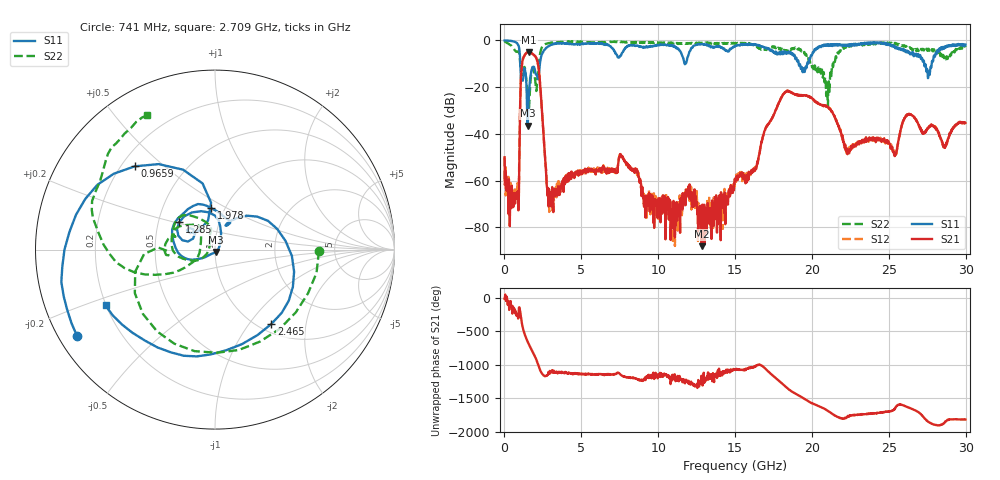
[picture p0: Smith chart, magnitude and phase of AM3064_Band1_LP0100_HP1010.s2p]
# Hz S DB R 50.0
!freq dBS11 angS11 dBS21 angS21 dBS12 angS12 dBS22 angS22
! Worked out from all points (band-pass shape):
!   1600 points, 10 MHz to 29.98 GHz, reference 50 ohm
!   highest |S21| = -4.96 dB at 1.603 GHz (marker M1); lowest = -88.1 dB at 12.83 GHz (marker M2)
!   |S21| within 3 dB of the highest: 1.206 GHz to 2.093 GHz (887.7 MHz wide, 53.8 % of centre)
!   lowest |S11| = -36.5 dB at 1.51 GHz (marker M3), VSWR 1.03, Z = 50.7 - j1.35 ohm
!   |S11| at or under -10 dB: 1.031 GHz to 2.306 GHz (1.275 GHz wide, 76.4 % of centre); 19.14 GHz to 19.69 GHz (546.8 MHz wide, 2.82 % of centre); 27.3 GHz to 27.79 GHz (488.3 MHz wide, 1.77 % of centre)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
!   |S22| runs from -29.5 to -0.4 dB; largest |S21 - S12| = 0.0081
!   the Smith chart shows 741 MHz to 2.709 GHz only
!   S11 on the Smith chart (normalised r, x): 741 MHz: 0.05, -0.29; 965.9 MHz: 0.25, +0.40; 1.285 GHz: 0.64, +0.21; 1.978 GHz: 0.86, +0.42; 2.465 GHz: 1.14, -1.29; 2.709 GHz: 0.20, -0.23
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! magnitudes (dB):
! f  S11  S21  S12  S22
! 10 MHz  0.0  -50.0  -50.2  -0.4
! 741 MHz  -0.8  -66.3  -66.3  -4.7
! 965.9 MHz  -3.8  -49.1  -48.6  -5.9
! 1.285 GHz  -12.0  -6.7  -6.7  -11.4
! 1.51 GHz  -36.5  -5.0  -5.0  -22.8
! 1.603 GHz  -21.6  -5.0  -5.0  -28.6
! 1.978 GHz  -12.7  -6.6  -6.6  -15.8
! 2.465 GHz  -5.7  -32.6  -32.6  -2.7
! 2.709 GHz  -3.3  -57.3  -55.3  -1.5
! 3.065 GHz  -1.9  -66.3  -70.2  -1.0
! 5.015 GHz  -1.4  -56.4  -55.9  -0.6
! 7.601 GHz  -6.1  -49.4  -49.0  -0.7
! 10 GHz  -2.0  -70.4  -73.4  -1.0
! 12.83 GHz  -1.6  -88.1  -71.1  -1.1
! 15 GHz  -2.5  -60.1  -59.3  -1.3
! 18.21 GHz  -5.6  -22.5  -22.4  -4.3
! 19.99 GHz  -6.5  -24.8  -24.8  -10.8
! 21.02 GHz  -1.7  -28.5  -28.6  -26.1
! 22.28 GHz  -2.5  -46.4  -48.5  -2.3
! 25 GHz  -1.5  -44.1  -44.2  -1.2
! 27.56 GHz  -15.9  -37.3  -37.2  -3.7
! 29.98 GHz  -1.8  -35.4  -34.8  -2.9
